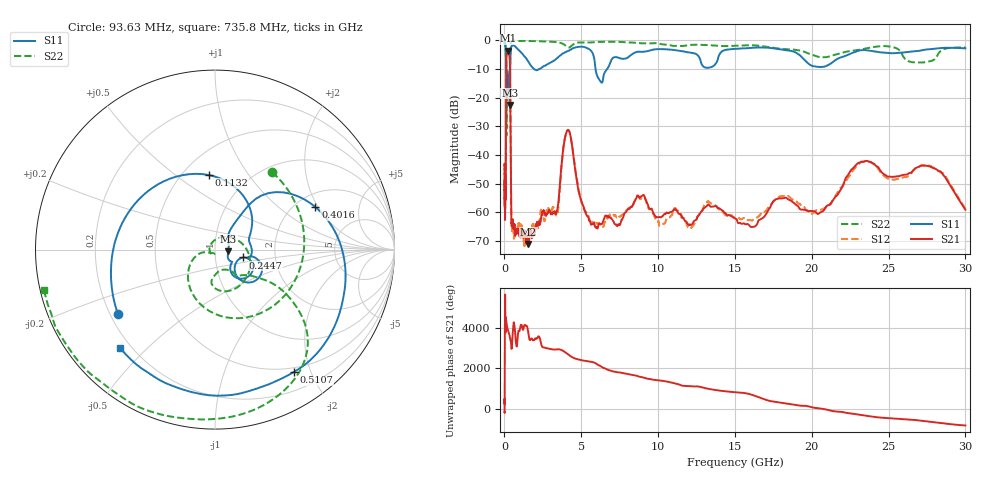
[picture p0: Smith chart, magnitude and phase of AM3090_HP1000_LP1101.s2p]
! Date/Time: Thu, Feb 28, 2019 2:02 PM
! Network Analyzer: Agilent Technologies E8364B Rev: A.07.50.67
! Sweep from 0.010 to 30.000 GHz, 1601 Points, Sweep Type: LOG
! Power Supply: 5.023 V, 0.002 A
# Hz S DB R 50
!freq MagS11 AngS11 MagS21 AngS21 MagS12 AngS12 MagS22 AngS22
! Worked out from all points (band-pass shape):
!   1601 points, 10 MHz to 30 GHz, reference 50 ohm
!   highest |S21| = -3.70 dB at 231.6 MHz (marker M1); lowest = -71.0 dB at 1.551 GHz (marker M2)
!   |S21| within 3 dB of the highest: 123.7 MHz to 347.6 MHz (223.9 MHz wide, 95 % of centre)
!   lowest |S11| = -22.5 dB at 340.5 MHz (marker M3), VSWR 1.16, Z = 58 - j1.12 ohm
!   |S11| at or under -10 dB: 118.3 MHz to 381 MHz (262.7 MHz wide, 105 % of centre); 1.895 GHz to 2.276 GHz (381.2 MHz wide, 18.3 % of centre); 5.925 GHz to 6.695 GHz (770.5 MHz wide, 12.2 % of centre)
!   |S22| runs from -33.3 to -0.1 dB; largest |S21 - S12| = 0.012
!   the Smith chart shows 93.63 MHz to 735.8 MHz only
!   S11 on the Smith chart (normalised r, x): 93.63 MHz: 0.23, -0.29; 113.2 MHz: 0.66, +0.67; 244.7 MHz: 1.37, -0.12; 401.6 MHz: 2.52, +1.89; 510.7 MHz: 0.44, -1.75; 735.8 MHz: 0.16, -0.42
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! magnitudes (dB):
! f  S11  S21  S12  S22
! 10 MHz  -0.2  -43.7  -48.9  -0.7
! 38.04 MHz  -0.5  -60.0  -60.5  -1.6
! 93.63 MHz  -3.8  -43.6  -42.9  -5.4
! 113.2 MHz  -7.6  -14.1  -14.1  -8.6
! 144.7 MHz  -14.0  -4.3  -4.3  -30.1
! 231.6 MHz  -17.2  -3.7  -3.7  -15.1
! 244.7 MHz  -15.7  -3.7  -3.7  -16.0
! 340.5 MHz  -22.5  -6.0  -6.0  -12.5
! 401.6 MHz  -4.3  -36.5  -36.2  -1.1
! 443.9 MHz  -2.4  -60.9  -60.8  -0.4
! 510.7 MHz  -1.8  -63.7  -66.2  -0.2
! 550.5 MHz  -1.8  -62.8  -64.4  -0.2
! 735.8 MHz  -2.4  -65.9  -66.0  -0.2
! 1.551 GHz  -7.5  -71.0  -67.3  -0.3
! 2.084 GHz  -10.5  -65.1  -63.9  -0.4
! 3.402 GHz  -6.4  -59.7  -60.9  -0.7
! 4.115 GHz  -3.8  -31.4  -31.3  -2.5
! 5.528 GHz  -3.2  -63.0  -62.2  -0.8
! 7.926 GHz  -6.3  -59.8  -59.3  -0.8
! 15.97 GHz  -2.8  -64.8  -62.7  -1.8
! 23.48 GHz  -3.5  -42.1  -42.4  -3.0
! 30 GHz  -2.8  -59.1  -58.8  -2.5
